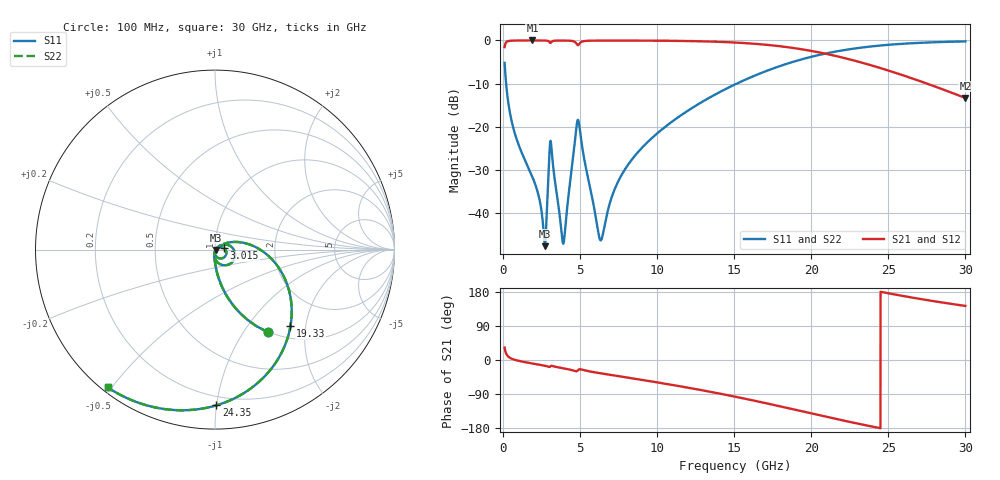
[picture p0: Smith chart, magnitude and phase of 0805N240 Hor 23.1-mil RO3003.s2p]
# GHz S MA R 50
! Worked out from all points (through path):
!   3201 points, 100 MHz to 30 GHz, reference 50 ohm
!   highest |S21| = -0.02 dB at 1.903 GHz (marker M1); lowest = -13.4 dB at 30 GHz (marker M2)
!   group delay of S21, straight-line fit = 21.5 ps
!   lowest |S11| = -47.7 dB at 2.716 GHz (marker M3), VSWR 1.01, Z = 50.4 - j0.217 ohm
!   |S11| at or under -10 dB: 196.7 MHz to 15.18 GHz (14.98 GHz wide, 195 % of centre)
!   |S22| runs from -47.7 to -0.2 dB; largest |S21 - S12| = 0
!   S11 on the Smith chart (normalised r, x): 100 MHz: 0.99, -1.31; 3.015 GHz: 1.11, +0.02; 19.33 GHz: 1.23, -1.65; 24.35 GHz: 0.14, -1.00; 30 GHz: 0.02, -0.49
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0.1  0.5488 -57.2  0.8355 32.7  0.8355 32.7  0.5488 -57.2
0.32425  0.1976 -80.3  0.9798 9.6  0.9798 9.6  0.1976 -80.3
0.6699688  0.09543 -87.9  0.9947 1.7  0.9947 1.7  0.09543 -87.9
1.903344  0.02609 -96.2  0.9982 -9.2  0.9982 -9.2  0.02609 -96.2
2.305125  0.01587 -95.7  0.998 -12.1  0.998 -12.1  0.01587 -95.7
2.71625  0.004106 -31.7  0.996 -15.2  0.996 -15.2  0.004106 -31.7
2.809687  0.007984 23.0  0.9937 -16.1  0.9937 -16.1  0.007984 23.0
3.01525  0.05168 8.5  0.9535 -18.3  0.9535 -18.3  0.05168 8.5
3.174094  0.0479 -71.0  0.9719 -15.6  0.9719 -15.6  0.0479 -71.0
3.902906  0.004383 -26.3  0.9955 -21.9  0.9955 -21.9  0.004383 -26.3
4.771875  0.1025 1.7  0.9109 -29.7  0.9109 -29.7  0.1025 1.7
4.912031  0.1128 -47.5  0.8947 -24.9  0.8947 -24.9  0.1128 -47.5
5.089563  0.06649 -81.9  0.9618 -25.2  0.9618 -25.2  0.06649 -81.9
6.341625  0.00479 -28.9  0.995 -35.2  0.995 -35.2  0.00479 -28.9
7.631062  0.02632 37.8  0.9954 -43.5  0.9954 -43.5  0.02632 37.8
10.06978  0.08545 27.6  0.9917 -59.5  0.9917 -59.5  0.08545 27.6
15.05  0.3085 -7.9  0.9445 -96.7  0.9445 -96.7  0.3085 -7.9
19.32944  0.5995 -45.5  0.7914 -134.7  0.7914 -134.7  0.5995 -45.5
20.03956  0.6475 -52.0  0.7527 -141.3  0.7527 -141.3  0.6475 -52.0
24.34703  0.8677 -89.5  0.486 -178.8  0.486 -178.8  0.8677 -89.5
25.01978  0.8893 -94.7  0.446 175.9  0.446 175.9  0.8893 -94.7
30  0.9734 -127.9  0.2148 142.7  0.2148 142.7  0.9734 -127.9
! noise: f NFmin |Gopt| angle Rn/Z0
0.1  0.0005657  0.892  0.8114  0.00114
3.417  0.01114  0.8209  19.2  0.01269
6.743  0.01277  0.7157  37.29  0.007992
10.06  0.01553  0.6704  54.19  0.007253
13.39  0.02014  0.6729  69.93  0.008113
16.7  0.02603  0.692  84.48  0.009273
20.03  0.03392  0.7226  98.16  0.01076
23.35  0.04505  0.762  111.2  0.01274
26.67  0.06198  0.8083  124  0.01543
30  0.08992  0.8577  136.8  0.01902
